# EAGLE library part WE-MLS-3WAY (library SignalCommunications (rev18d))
Multiline EMI Suppression Ferrite Characteristics High impedance common mode inductor with 2x2 windings made by PCB line connection High rated current with typ. 4 A Broadband filtering because of the NiZn-ferrite core RF common mode inductor for 2, 3 or 4 lines in one component Compact size Operating temperature: –25 ºC to +125 ºC Custom designs on request With the appropriate layout (see below) the impedance (i.e. 4 windings) respectively the current (parallel circuit) could be increased Applications Perfect suitable for absorption of common or differential mode interferences in the field of EMC High-current DC output filters of power supplies e.g. battery chargers, industrial power supplies With one turn the component performes like a 3 or 4 times common mode choke for the signal 4-line sensor application Details see: http://katalog.we-online.de/en/pbs/WE-MLS? Updated by Dan Xu 2014-07-08 2014 (C) Wurth Elektronik
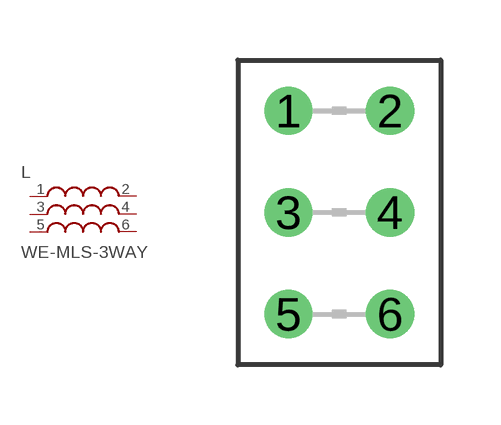
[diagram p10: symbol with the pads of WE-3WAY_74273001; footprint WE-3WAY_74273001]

Designator prefix L

## WE-MLS-3WAY_74273001  [WE-3WAY_74273001]
1  1  pas
2  2  pas
3  3  pas
4  4  pas
5  5  pas
6  6  pas

## Footprint WE-3WAY_74273001 (pad centres in mm)
Multiline EMI Suppression Ferrite WE-MLS
drill 0.7: 1 -1.27,2.54; 2 1.27,2.54; 3 -1.27,0; 4 1.27,0; 5 -1.27,-2.54; 6 1.27,-2.54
